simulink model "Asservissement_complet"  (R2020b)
settings: Solver=FixedStepAuto  StartTime=0.0  StopTime=inf  FixedStep=0.01  RelTol=1e-3  EnableMultiTasking=on
libraries: arduinolib x5, simulink x1, pid_lib x1

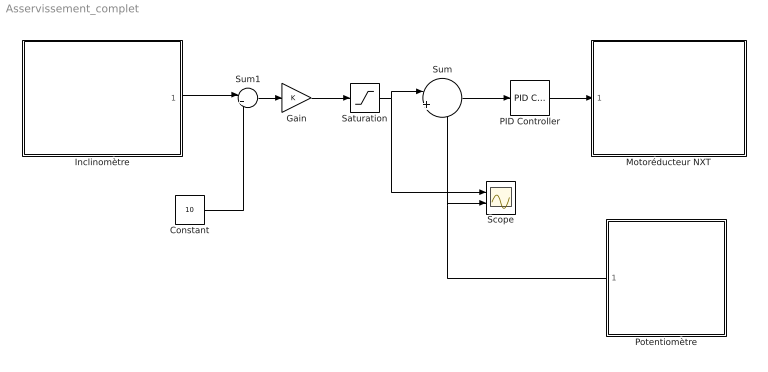
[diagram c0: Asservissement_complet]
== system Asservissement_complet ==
  Constant : Constant  Value=10
  Gain : Gain
  Inclinomètre : Subsystem
  Motoréducteur NXT : Subsystem
  PID Controller : pid_lib/PID Controller  Controller=PID  Form=Parallel  TimeDomain=Discrete-time  UseExternalTs=off  SampleTime=-1  IntegratorMethod=Forward Euler  FilterMethod=Forward Euler  ControllerParametersSource=internal  P=0.1  I=0  D=0  UseFilter=on  N=100  TunerSelectOption=Transfer Function Based (PID Tuner App)  InitialConditionSource=internal  InitialConditionForIntegrator=0  InitialConditionForFilter=0  DifferentiatorICPrevScaledInput=0  ExternalReset=none  TrackingMode=off  Kt=1  LimitOutput=off  SatLimitsSource=internal  UpperSaturationLimit=inf  LowerSaturationLimit=-inf  LinearizeAsGain=on  AntiWindupMode=none  Kb=1  POutMin=[]  POutMax=[]  IOutMin=[]  IOutMax=[]  DOutMin=[]  DOutMax=[]  NOutMin=[]  NOutMax=[]  SumOutMin=[]  SumOutMax=[]  SaturationOutMin=[]  SaturationOutMax=[]  PParamMin=[]  PParamMax=[]  IParamMin=[]  IParamMax=[]  DParamMin=[]  DParamMax=[]  NParamMin=[]  NParamMax=[]  KbParamMin=[]  KbParamMax=[]  KtParamMin=[]  KtParamMax=[]  KbOutMin=[]  KbOutMax=[]  KtOutMin=[]  KtOutMax=[]  IntegratorOutMin=[]  IntegratorOutMax=[]  FilterOutMin=[]  FilterOutMax=[]  SumI1OutMin=[]  SumI1OutMax=[]  SumI2OutMin=[]  SumI2OutMax=[]  SumI3OutMin=[]  SumI3OutMax=[]  SumI4OutMin=[]  SumI4OutMax=[]  SumDOutMin=[]  SumDOutMax=[]  DifferentiatorOutMin=[]  DifferentiatorOutMax=[]  FilterDiffOutCoefMin=[]  FilterDiffOutCoefMax=[]  ReciprocalOutMin=[]  ReciprocalOutMax=[]  SumDenOutMin=[]  SumDenOutMax=[]  SumNumOutMin=[]  SumNumOutMax=[]  DivideOutMin=[]  DivideOutMax=[]  UdiffTsProdOutMin=[]  UdiffTsProdOutMax=[]  NTsProdOutMin=[]  NTsProdOutMax=[]  UintegralTsProdOutMin=[]  UintegralTsProdOutMax=[]  UngainTsProdOutMin=[]  UngainTsProdOutMax=[]  IntegratorContinuousStateAttributes=''  IntegratorStateMustResolveToSignalObject=off  IntegratorRTWStateStorageClass=Auto  FilterContinuousStateAttributes=''  FilterStateMustResolveToSignalObject=off  FilterRTWStateStorageClass=Auto  ParallelPVariant=InternalParameters  IdealPVariant=Disabled  IVariant=InternalParameters  DVariant=InternalParameters  IntegratorVariant=Discrete  SatVariant=Disabled  AWVariant=Passthrough  PCopyVariant=Disabled  TRVariant=Disabled  FdbkBlocksVariant=Forward  IdealPFdbkVariant=Disabled  SatFdbkVariant=Disabled  DerivativeFilterVariant=ForwardEulerFilter  NVariant=InternalParameters  NCopyVariant=Disabled  FilterICVariant=InternalICsFilter  IntegratorICVariant=InternalICs  ExternalResetVariant=Disabled  TRSumVariant=Passthrough  SumFdbkVariant=Disabled  SumVariant=Sum_PID  TsampFilterVariant=InternalTs  TsampNgainVariant=Passthrough  TsampIntegralVariant=Passthrough  ExternalSaturationOutDataTypeStr=Inherit: Same as second input
  Potentiomètre : Subsystem
  Saturation : Saturate  UpperLimit=150  LowerLimit=10
  Scope : Scope  NumInputPorts=2
  Sum : Sum  Inputs=|+-
  Sum1 : Sum  Inputs=|++
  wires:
  Potentiomètre/1(Out1) -> Scope/2, Sum/2
  Sum/1 -> PID Controller/1
  PID Controller/1 -> Motoréducteur NXT/1(U)
  Sum1/1 -> Gain/1
  Inclinomètre/1(d) -> Sum1/1
  Constant/1 -> Sum1/2
  Gain/1 -> Saturation/1
  Saturation/1 -> Scope/1, Sum/1

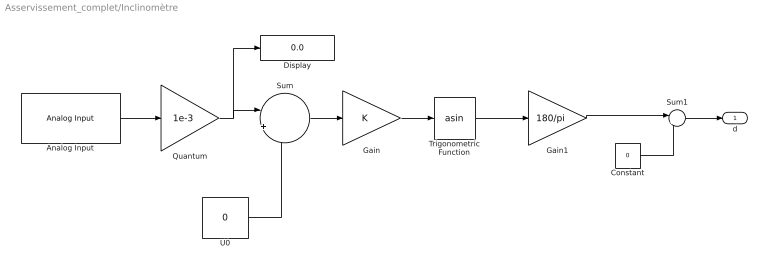
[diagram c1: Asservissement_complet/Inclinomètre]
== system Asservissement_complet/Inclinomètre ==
  Analog Input : arduinolib/Analog Input  pinNumber=2  ReadResultsOnly=off  ConversionTriggerSource=Software  ExternalTriggerType=uint32(0)  OutputDataType=uint16  EnableConversionCompleteNotify=off  EnableOuputStatus=off  SampleTime=0.01  blockPlatform=arduino
  Constant : Constant  Value=0
  Display : Display
  Gain : Gain
  Gain1 : Gain  Gain=180/pi
  Quantum : Gain  Gain=1e-3
  Sum : Sum  Inputs=|+-
  Sum1 : Sum  Inputs=|++
  Trigonometric Function : Trigonometry  Operator=asin
  U0 : Constant  Value=0
  d : Outport  VectorParamsAs1DForOutWhenUnconnected=off
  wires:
  Gain/1 -> Trigonometric Function/1
  Sum1/1 -> d/1
  Trigonometric Function/1 -> Gain1/1
  Analog Input/1 -> Quantum/1
  U0/1 -> Sum/2
  Quantum/1 -> Display/1, Sum/1
  Sum/1 -> Gain/1
  Gain1/1 -> Sum1/1
  Constant/1 -> Sum1/2

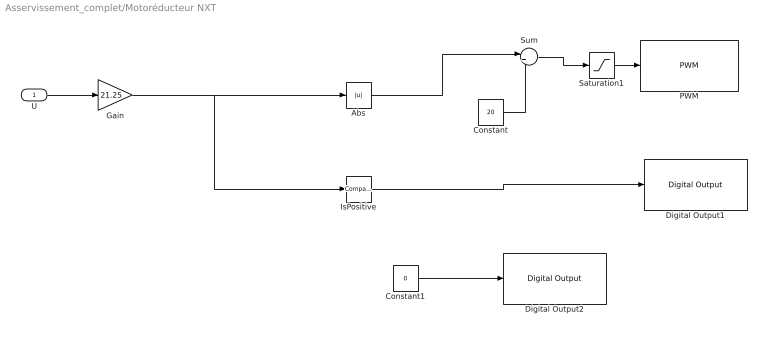
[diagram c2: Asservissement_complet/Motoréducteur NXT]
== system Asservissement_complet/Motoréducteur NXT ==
  U : Inport
  Abs : Abs
  Constant : Constant  Value=20
  Constant1 : Constant  Value=0
  Digital Output1 : arduinolib/Digital Output  pinNumber=12  Direction=output  blockPlatform=arduino
  Digital Output2 : arduinolib/Digital Output  pinNumber=9  Direction=output  blockPlatform=arduino
  Gain : Gain  Gain=21.25
  IsPositive : simulink/Logic and Bit Operations/Compare To Zero  relop=>  OutDataTypeStr=boolean
  PWM : arduinolib/PWM  pinNumber=3  frequencyType=Default  desiredFrequency=490.2  achievableFrequency=490.2
  Saturation1 : Saturate  UpperLimit=255  LowerLimit=0
  Sum : Sum  Inputs=|++
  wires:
  U/1 -> Gain/1
  Constant1/1 -> Digital Output2/1
  Sum/1 -> Saturation1/1
  Saturation1/1 -> PWM/1
  Constant/1 -> Sum/2
  IsPositive/1 -> Digital Output1/1
  Abs/1 -> Sum/1
  Gain/1 -> Abs/1, IsPositive/1

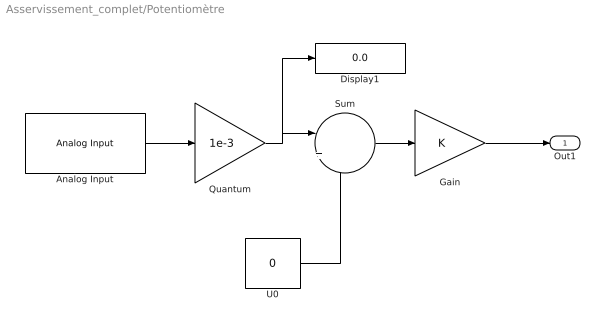
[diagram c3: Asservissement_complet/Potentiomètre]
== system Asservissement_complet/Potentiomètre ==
  Analog Input : arduinolib/Analog Input  pinNumber=0  ReadResultsOnly=off  ConversionTriggerSource=Software  ExternalTriggerType=uint32(0)  OutputDataType=uint16  EnableConversionCompleteNotify=off  EnableOuputStatus=off  SampleTime=0.01  blockPlatform=arduino
  Display1 : Display
  Gain : Gain
  Quantum : Gain  Gain=1e-3
  Sum : Sum  Inputs=|+-
  U0 : Constant  Value=0
  Out1 : Outport  VectorParamsAs1DForOutWhenUnconnected=off
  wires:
  Gain/1 -> Out1/1
  Analog Input/1 -> Quantum/1
  Quantum/1 -> Display1/1, Sum/1
  U0/1 -> Sum/2
  Sum/1 -> Gain/1
